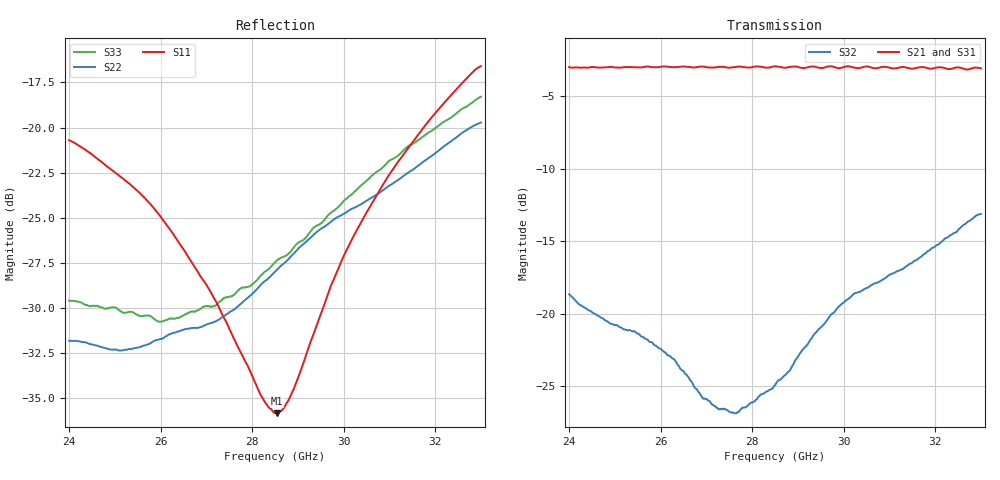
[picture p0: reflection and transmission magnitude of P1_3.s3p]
!The following data was pulled from an Agilent PNA
!This sNp file was generated from the data in the RF Test software
!NOTE:  Smoothing/Math/Corrections applied on any given trace ARE included in the data saved here
# MHz S dB R 50
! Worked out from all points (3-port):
!   1601 points, 24 GHz to 33 GHz, reference 50 ohm
!   strongest paths, dB at 24 GHz, 26.25 GHz, 28.5 GHz, 30.75 GHz, 33 GHz:
!     S21: -3.0, -3.0, -3.0, -3.1, -3.1
!     S31: -3.0, -3.0, -3.1, -3.2, -3.3
!     S32: -18.7, -23.1, -24.9, -17.8, -13.1
!   lowest |S11| = -35.8 dB at 28.54 GHz (marker M1), VSWR 1.03, Z = 50.4 + j1.57 ohm
!   |S11| at or under -10 dB: start of sweep to end of sweep
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24000  -20.70 30.2  -3.13 153.7  -3.09 152.7
       -3.01 153.7  -31.80 -159.7  -18.65 99.2
       -2.99 152.2  -18.65 98.8  -29.59 178.4
25777.5  -24.24 20.0  -3.10 136.4  -3.07 135.1
         -2.99 136.3  -31.94 -174.0  -21.94 67.2
         -3.00 135.0  -21.95 66.8  -30.45 155.7
27251.25  -29.83 21.5  -3.06 121.7  -3.07 120.0
          -3.00 121.7  -30.66 170.6  -26.51 19.5
          -3.06 119.5  -26.53 19.2  -29.73 146.2
27673.12  -32.07 28.9  -3.04 117.3  -3.09 115.6
          -2.97 117.5  -29.94 168.2  -26.76 5.7
          -3.10 115.2  -26.80 5.4  -29.07 143.9
28500  -35.81 71.8  -3.05 108.7  -3.13 107.0
       -2.96 108.9  -27.98 160.9  -24.89 -30.2
       -3.14 106.9  -24.91 -30.4  -27.47 140.6
28539.38  -35.82 74.9  -3.04 108.3  -3.13 106.6
          -2.96 108.3  -27.88 160.4  -24.69 -31.9
          -3.14 106.6  -24.71 -32.1  -27.36 140.4
28927.5  -34.36 102.0  -3.04 104.2  -3.15 102.5
         -2.96 104.4  -26.93 155.9  -23.29 -45.5
         -3.16 102.5  -23.29 -45.7  -26.59 137.5
29895  -27.73 130.8  -3.06 94.0  -3.20 92.4
       -3.08 94.4  -24.92 142.0  -19.47 -80.8
       -3.13 92.5  -19.51 -81.2  -24.36 130.1
30530.62  -24.58 133.6  -3.06 87.3  -3.23 85.9
          -2.97 87.4  -24.01 134.3  -18.18 -98.7
          -3.27 86.1  -18.20 -98.9  -22.88 123.3
33000  -16.60 121.2  -3.21 60.1  -3.37 59.1
       -3.09 60.6  -19.72 109.8  -13.05 -139.3
       -3.31 59.7  -13.12 -139.5  -18.29 97.2
